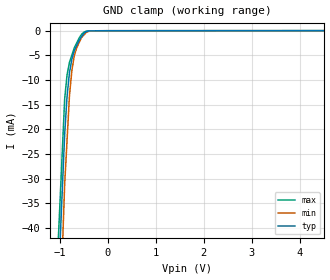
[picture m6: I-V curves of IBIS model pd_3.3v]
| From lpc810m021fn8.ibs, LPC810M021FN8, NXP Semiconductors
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[Model] pd_3.3v
Model_type Input
Vinl = 990.000mV
Vinh = 2.31000V
C_comp 587.000fF 585.000fF 589.000fF
| variable typ   min   max
[Voltage Range] 3.30000V 3.00000V 3.60000V
[POWER Clamp Reference] 3.30000V 3.00000V 3.60000V
[GND Clamp Reference] 0.00000V 0.00000V 0.00000V
[Temperature Range]   25   85   -40
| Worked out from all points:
|   GND clamp passes 1 mA (typ) near -0.53 V on its own axis
[GND Clamp]
-3.3V     -567.9mA   -692.8mA   -529.3mA
-900mV    -20.98mA   -31.13mA   -13.8mA
-850mV    -13.28mA   -22.15mA   -8.911mA
-800mV    -8.483mA   -13.16mA   -6.412mA
-750mV    -5.729mA   -8.059mA   -4.946mA
-700mV    -4.056mA   -5.078mA   -3.479mA
-650mV    -2.988mA   -3.465mA   -2.487mA
-600mV    -1.919mA   -2.438mA   -1.496mA
-550mV    -1.226mA   -1.411mA   -758.6uA
-450mV    -189.9uA   -355.1uA   -86.11uA
-200mV    -8.97uA    -6.932uA   -21.03uA
6.6V      13.29uA    12.58uA    30.09uA
[POWER Clamp]
-3.3V     0A         0A         0A
6.6V      0A         0A         0A
